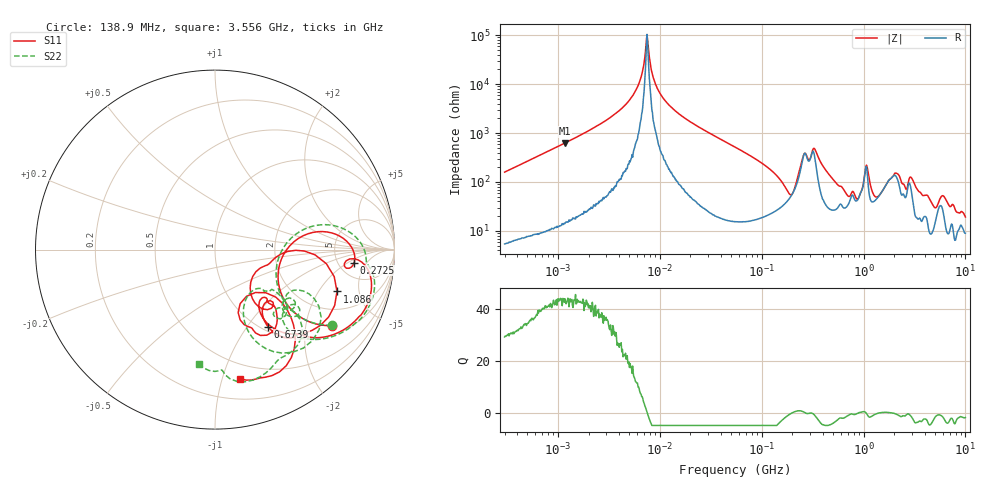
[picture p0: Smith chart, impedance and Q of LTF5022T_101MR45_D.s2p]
! S-Parameter Data Generated by TDK Corporation
! Copyright(C) 2020 TDK Corporation.
! All Rights Reserved.
! TDK P/N: LTF5022T-101MR45-D (Inductor)
! Property: L=100uH at 100kHz
! Size(LxWxT): 6.5x5x2.2mm
! Model Type: s2p (Touchstone File Format Version 1.0)
! Frequency: DC=Yes Start=0.3MHz Stop=10000MHz 802points Log-sweep
! Model Generated on Apr. 23, 2020
! Port Assignments:
!  1 ---@@@--- 2
! Applicable Conditions:
!  Temperature = 25 degC
!  DC Bias Current = 0 A
!  Small Signal Operation
! Terms and conditions regarding TDK Simulation Models
! (1)This simulation model is being provided solely for informational purposes. Please refer to the specifications of the products in terms of detailed characteristics of such products.
! (2)In no event shall TDK Corporation of any of its subsidiaries be liable for any loss or damage arising, directly or indirectly,
!  From any information contained in this simulation model, including, but not limited to loss or damages arising from any inaccuracies, omissions or errors in connection with such information.
! (3)Any and all copyrights on this simulation model are owned by TDK Corporation.
!  Duplication or redistribution of this simulation model without prior written permission from TDK Corporation is prohibited.
! (4)This simulation model is subject to any modification or change without any prior notice.
! (5)Neither TDK Corporation nor any of its subsidiaries shall make any warranty, express or implied,
!  Including but not limited to the correctness, implied warranties of merchantability and fitness for a particular purpose with respect to this simulation models.
! (6)The use of this simulation model shall be deemed to have consented to the terms and conditions hereof.
# Hz S MA R 50
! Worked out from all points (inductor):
!   801 points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, 300 kHz to 10 GHz, reference 50 ohm
!   read as 1/Y11, port 2 shorted: L = 83.9 uH near 318.3 kHz
!   highest Q = 44 at 1.17 MHz (marker M1), where L = 84.7 uH
!   self-resonance near 7.5 MHz
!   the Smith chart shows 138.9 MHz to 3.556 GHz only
!   S11 on the Smith chart (normalised r, x): 138.9 MHz: 1.32, -2.82; 272.5 MHz: 7.08, -2.60; 673.9 MHz: 1.07, -1.27; 1.086 GHz: 3.08, -2.97; 3.556 GHz: 0.37, -1.15
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300000  0.8338 31.6  0.5244 -56.5  0.5244 -56.4  0.8333 31.6
1170165  0.9838 9.1  0.1581 -79.7  0.1582 -79.7  0.9837 9.1
1713600  0.9918 6.1  0.1067 -82.7  0.1067 -82.7  0.9917 6.1
5354396  0.9986 1.0  0.02074 -86.0  0.02071 -86.3  0.9986 1.0
8128066  0.999 -0.2  0.000979 -14.2  0.0009302 -9.6  0.9989 -0.2
9671944  0.9989 -0.8  0.00818 81.8  0.008178 81.8  0.9988 -0.7
5.477226e7  0.9814 -10.9  0.1604 77.2  0.1604 77.2  0.9814 -10.8
1.389026e8  0.7768 -33.0  0.4914 45.3  0.4914 45.3  0.776 -32.8
1.945824e8  0.3732 -19.1  0.6474 1.3  0.6474 1.3  0.3595 -18.5
2.725454e8  0.7791 -5.3  0.2099 -33.3  0.2091 -33.3  0.8293 0.4
3.126428e8  0.7988 -4.1  0.1501 -23.4  0.1504 -23.1  0.8824 -7.8
6.738867e8  0.5226 -55.5  0.5849 9.2  0.5845 9.2  0.5564 -41.8
1.085776e9  0.7184 -18.9  0.2466 -26.6  0.2473 -26.5  0.7431 -42.8
1.767019e9  0.3949 -43.4  0.6086 -57.8  0.6088 -57.8  0.3463 -39.8
2.69003e9  0.3139 -56.0  0.3011 -99.1  0.3019 -99.0  0.6875 -45.6
3.556288e9  0.7323 -78.9  0.1806 -114.0  0.1797 -114.2  0.6445 -98.1
4.166115e9  0.6467 -84.9  0.2675 -147.0  0.2645 -146.0  0.4737 -80.6
4.982529e9  0.6686 -120.4  0.03114 -104.3  0.02769 -112.6  0.6656 -94.8
6.010849e9  0.5615 -90.6  0.2205 -124.4  0.22 -123.1  0.7578 -101.3
7.652089e9  0.776 -113.3  0.01216 -161.8  0.01123 -170.8  0.8016 -120.3
8.658336e9  0.6518 -134.9  0.1949 -165.3  0.1947 -163.3  0.6276 -118.9
1e10  0.7365 -140.9  0.1031 97.0  0.1056 97.2  0.7486 -127.0
